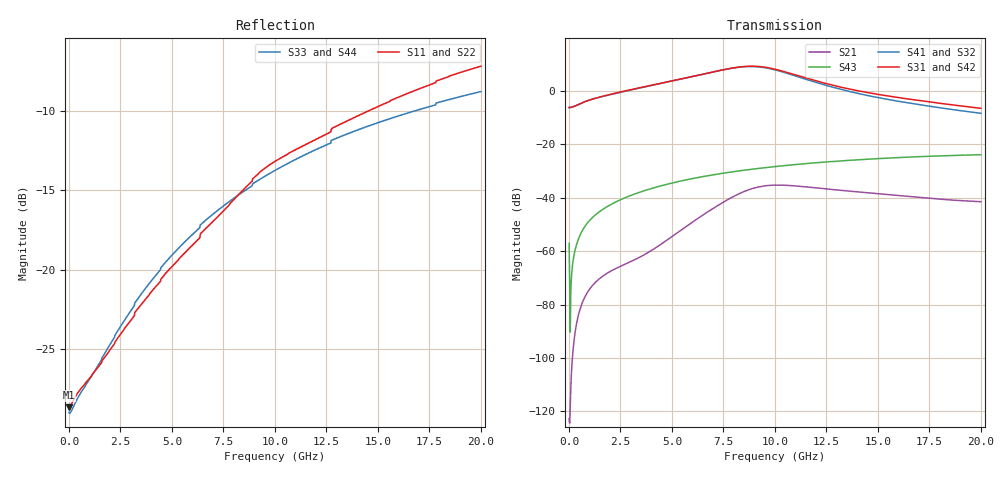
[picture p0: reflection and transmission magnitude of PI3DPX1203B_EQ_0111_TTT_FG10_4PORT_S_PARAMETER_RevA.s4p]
! NPort=4 DATA=2000 NOISE=0 GROUPDELAY=0 COMPLEX_DATAFORMAT=POLAR
! NumOfBlock=1 NumOfParam=0
! .MODEL Smodel S TSTONEFILE=PI3DPX1203B_EQ_0111_TTT_FG10_4PORT_S_PARAMETER_RevA.s4p TYPE=S
!  -- The above .MODEL line can be used for the S element in the netlist.
! The s parameter is extracted from the linear redriver, it is not bi-directional; only s(4,1)s(4,2) and s(3,1)s(3,2)
! should be the insertion loss
!Port definition:
!Port1 = input+
!Port2 = input-
!Port3 = output+
!Port4 = output-
# Hz S MA R  50
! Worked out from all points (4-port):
!   2000 points, 10 MHz to 20 GHz, reference 50 ohm
!   strongest paths, dB at 10 MHz, 5.01 GHz, 10.01 GHz, 15.01 GHz, 20 GHz:
!     S31: -6.2, 3.8, 8.2, -1.3, -6.5
!     S42: -6.2, 3.8, 8.2, -1.3, -6.5
!     S41: -6.2, 3.8, 7.9, -2.5, -8.3
!     S32: -6.2, 3.8, 7.9, -2.5, -8.3
!     S43: -57.1, -34.4, -28.3, -25.3, -23.8
!     S21: -122.7, -54.5, -35.2, -38.4, -41.4
!   lowest |S11| = -28.6 dB at 10 MHz (marker M1), VSWR 1.08, Z = 46.4 - j0.0306 ohm
!   |S11| at or under -10 dB: start of sweep to 14.54 GHz
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1e7  0.03701 -179.5  7.338e-07 10.6  0 0.0  0 0.0
     7.338e-07 10.6  0.03701 -179.5  0 0.0  0 0.0
     0.4917 -0.1  0.4917 179.9  0.03566 178.2  0.001403 -77.8
     0.4917 179.9  0.4917 -0.1  0.001403 -77.8  0.03566 178.2
1.55e9  0.05074 -145.1  0.0003216 117.3  4.816e-12 73.9  4.559e-11 115.2
        0.0003216 117.3  0.05074 -145.1  4.559e-11 115.2  4.816e-12 73.9
        0.7827 9.9  0.7759 -170.1  0.05178 -142.4  0.005752 82.9
        0.7759 -170.1  0.7827 9.9  0.005752 82.9  0.05178 -142.4
6.03e9  0.1203 -110.8  0.003583 147.9  1.555e-08 -119.1  1.377e-07 67.1
        0.003582 147.9  0.1203 -110.8  1.376e-07 67.1  1.556e-08 -119.1
        1.879 -43.2  1.877 138.6  0.1297 -117.0  0.0231 65.0
        1.878 138.6  1.879 -43.2  0.0231 65.0  0.1297 -117.0
8.41e9  0.177 -105.4  0.01269 109.2  3.645e-07 156.6  1.007e-06 17.8
        0.01269 109.2  0.177 -105.4  1.005e-06 17.8  3.646e-07 156.6
        2.861 -100.0  2.831 81.4  0.1753 -115.9  0.03262 52.8
        2.832 81.4  2.86 -100.0  0.03262 52.8  0.1753 -115.9
9.9e9  0.2175 -107.2  0.01728 65.9  1.185e-06 95.1  2.018e-06 -19.7
       0.01727 66.0  0.2175 -107.2  2.015e-06 -19.6  1.186e-06 95.2
       2.621 -148.9  2.55 32.4  0.2039 -116.2  0.03813 44.9
       2.552 32.4  2.619 -148.9  0.03813 44.9  0.2039 -116.2
1.207e10  0.2588 -109.0  0.01532 24.4  2.989e-06 30.1  3.765e-06 -47.5
          0.0153 24.5  0.2588 -109.0  3.765e-06 -47.4  2.99e-06 30.2
          1.523 164.5  1.422 -13.8  0.2399 -117.5  0.04569 33.9
          1.423 -13.8  1.522 164.5  0.04569 33.9  0.2399 -117.5
2e10  0.4373 -117.2  0.008429 -17.8  2.223e-05 -108.0  3.18e-05 -133.9
      0.008468 -17.7  0.4373 -117.2  3.188e-05 -133.8  2.225e-05 -107.9
      0.4745 78.5  0.3833 -87.0  0.3637 -123.9  0.06431 -7.1
      0.383 -87.1  0.4751 78.5  0.06431 -7.1  0.3637 -123.9
